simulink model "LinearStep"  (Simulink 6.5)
settings: Solver=ode45  SolverMode=SingleTasking  StartTime=0.0  StopTime=5.0  RelTol=1e-3  AbsTol=1e-6

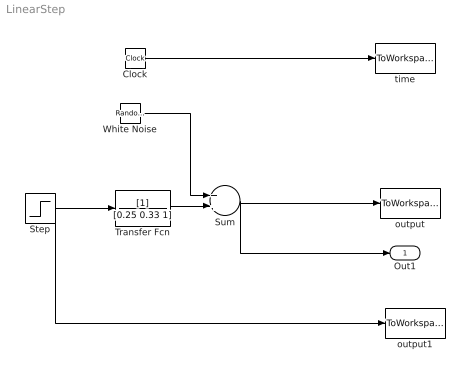
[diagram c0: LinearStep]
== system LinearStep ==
  Clock : Clock
  Step : Step  SampleTime=0.01
  Sum : Sum
  Transfer Fcn : TransferFcn  Denominator=[0.25 0.33 1]
  White Noise : RandomNumber  Variance=0.01  Seed=795  SampleTime=0.01
  output : ToWorkspace  VariableName=y  SampleTime=0.01  SaveFormat=Array
  output1 : ToWorkspace  VariableName=u  SampleTime=0.01  SaveFormat=Array
  time : ToWorkspace  VariableName=t  SampleTime=0.01  SaveFormat=Array
  Out1 : Outport
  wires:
  Step/1 -> Transfer Fcn/1, output1/1
  Transfer Fcn/1 -> Sum/2
  Clock/1 -> time/1
  Sum/1 -> output/1, Out1/1
  White Noise/1 -> Sum/1
